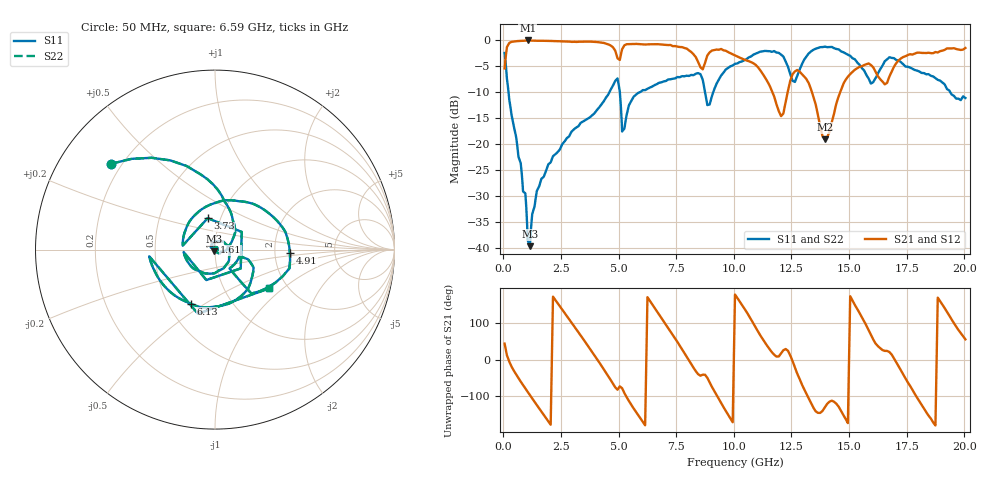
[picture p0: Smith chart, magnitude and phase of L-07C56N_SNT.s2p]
#	mhz	s	ma	r	50
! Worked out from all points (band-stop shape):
!   1001 points, 50 MHz to 20.05 GHz, reference 50 ohm
!   highest |S21| = -0.08 dB at 1.05 GHz (marker M1); lowest = -19.1 dB at 13.95 GHz (marker M2)
!   |S21| within 3 dB of the highest: 102.5 MHz to 4.923 GHz (4.82 GHz wide, 192 % of centre); 5.084 GHz to 8.311 GHz (3.227 GHz wide, 48.2 % of centre)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
!   lowest |S11| = -39.6 dB at 1.15 GHz (marker M3), VSWR 1.02, Z = 49.5 - j0.933 ohm
!   |S11| at or under -10 dB: 220.1 MHz to 4.6 GHz (4.38 GHz wide, 182 % of centre); 5.051 GHz to 5.929 GHz (877.7 MHz wide, 16 % of centre); 19.39 GHz to end of sweep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
!   |S22| runs from -39.6 to -1.3 dB; largest |S21 - S12| = 0
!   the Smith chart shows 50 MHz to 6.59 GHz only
!   S11 on the Smith chart (normalised r, x): 50 MHz: 0.16, +0.35; 1.61 GHz: 0.98, +0.09; 3.73 GHz: 0.87, +0.31; 4.91 GHz: 2.43, -0.12; 6.13 GHz: 0.65, -0.44; 6.59 GHz: 1.61, -0.81
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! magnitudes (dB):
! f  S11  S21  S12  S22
! 50 MHz  -2.5  -5.5  -5.5  -2.5
! 1.05 GHz  -38.5  -0.1  -0.1  -38.5
! 1.15 GHz  -39.6  -0.1  -0.1  -39.6
! 1.61 GHz  -27.2  -0.1  -0.1  -27.2
! 3.39 GHz  -15.8  -0.3  -0.3  -15.8
! 3.73 GHz  -14.9  -0.3  -0.3  -14.9
! 4.91 GHz  -7.6  -2.9  -2.9  -7.6
! 5.23 GHz  -17.1  -1.1  -1.1  -17.1
! 6.13 GHz  -9.6  -0.9  -0.9  -9.6
! 6.59 GHz  -8.6  -0.8  -0.8  -8.6
! 6.73 GHz  -8.3  -0.8  -0.8  -8.3
! 8.47 GHz  -6.4  -4.4  -4.4  -6.4
! 8.91 GHz  -12.4  -2.6  -2.6  -12.4
! 10.05 GHz  -4.6  -2.9  -2.9  -4.6
! 12.05 GHz  -2.8  -14.6  -14.6  -2.8
! 12.67 GHz  -7.8  -6.0  -6.0  -7.8
! 13.39 GHz  -2.1  -10.0  -10.0  -2.1
! 13.95 GHz  -1.3  -19.1  -19.1  -1.3
! 15.15 GHz  -3.5  -6.1  -6.1  -3.5
! 15.99 GHz  -8.3  -5.0  -5.0  -8.3
! 16.73 GHz  -3.4  -7.3  -7.3  -3.4
! 20.05 GHz  -11.1  -1.5  -1.5  -11.1
